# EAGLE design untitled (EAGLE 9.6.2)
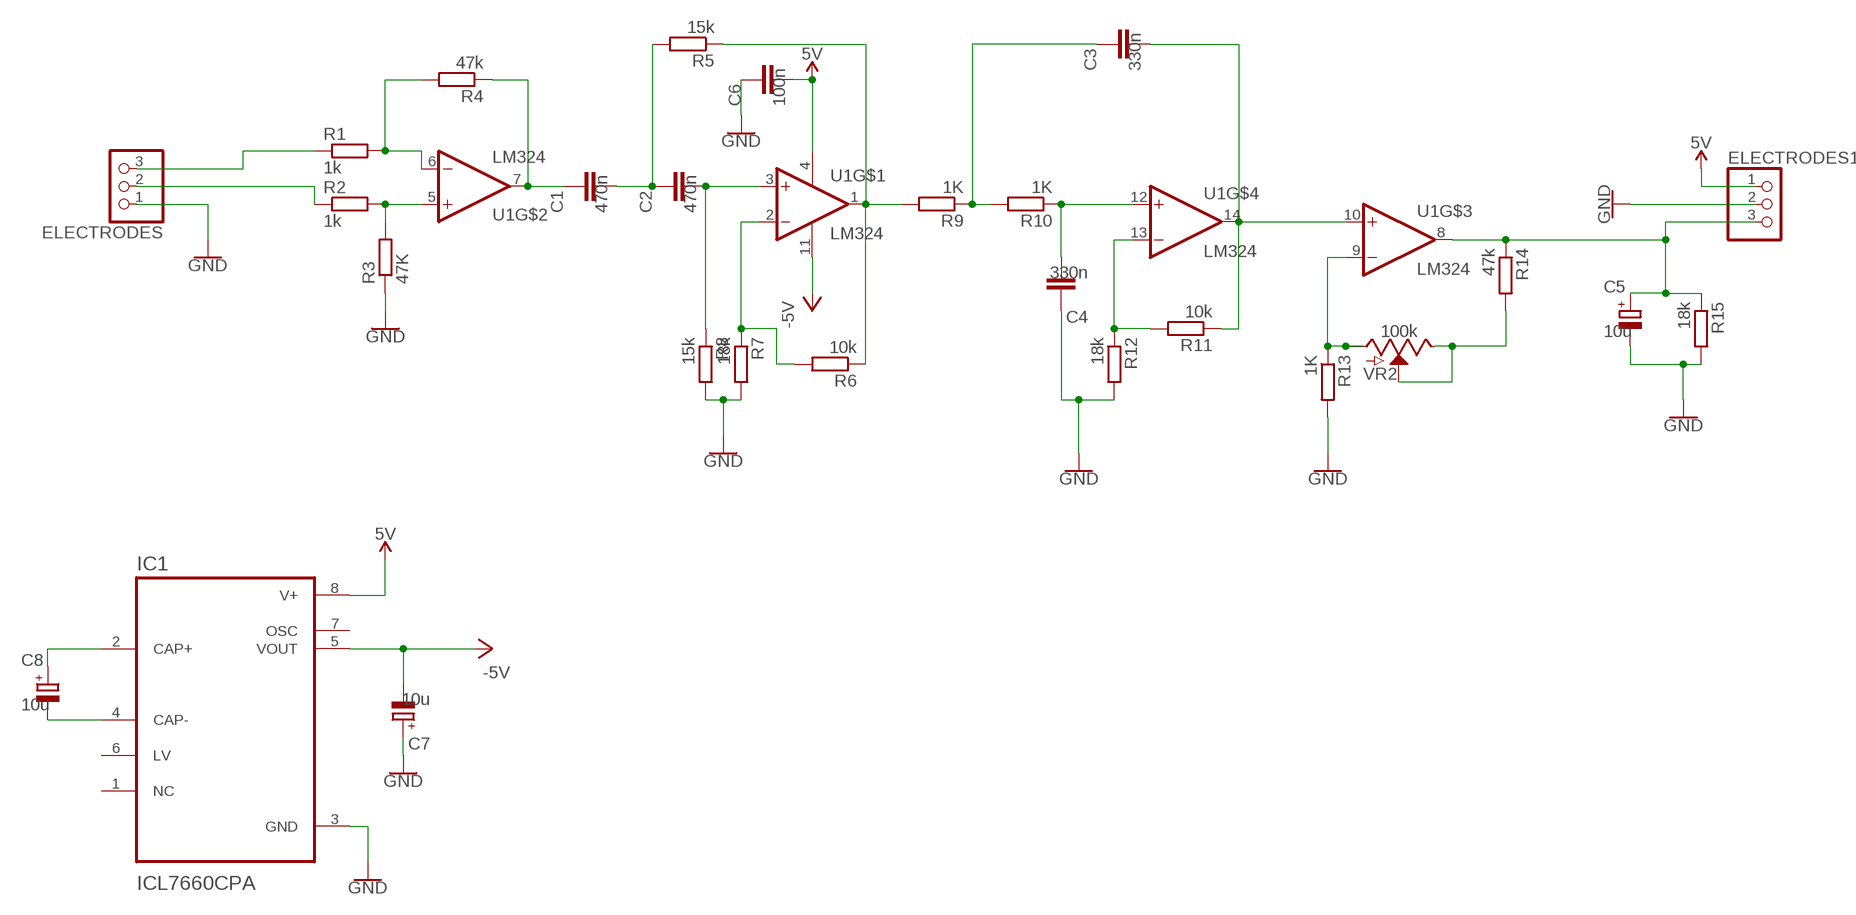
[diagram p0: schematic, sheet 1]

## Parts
C1  470n  C-EU025-024X044  [C025-024X044]
C2  470n  C-EU025-024X044  [C025-024X044]
C3  330n  C-EU025-024X044  [C025-024X044]
C4  330n  C-EU025-024X044  [C025-024X044]
C5  10u  CPOL-EUE2,5-6E  [E2,5-6E]
C6  100n  C-EU025-024X044  [C025-024X044]
C7  10u  CPOL-EUE2,5-6E  [E2,5-6E]
C8  10u  CPOL-EUE2,5-6E  [E2,5-6E]
ELECTRODES  PINHD-1X3  [1X03]
ELECTRODES1  PINHD-1X3  [1X03]
IC1  ICL7660CPA  [DIP794W47P254L991H457Q8]
R1  1k  R-EU_0204/7  [0204/7]
R2  1k  R-EU_0204/7  [0204/7]
R3  47K  R-EU_0204/7  [0204/7]
R4  47k  R-EU_0204/7  [0204/7]
R5  15k  R-EU_0204/7  [0204/7]
R6  10k  R-EU_0204/7  [0204/7]
R7  18k  R-EU_0204/7  [0204/7]
R8  15k  R-EU_0204/7  [0204/7]
R9  1K  R-EU_0204/7  [0204/7]
R10  1K  R-EU_0204/7  [0204/7]
R11  10k  R-EU_0204/7  [0204/7]
R12  18k  R-EU_0204/7  [0204/7]
R13  1K  R-EU_0204/7  [0204/7]
R14  47k  R-EU_0204/7  [0204/7]
R15  18k  R-EU_0204/7  [0204/7]
U1  LM324  [SOIC127P600X175-14N]
VR2  100k  POTENTIOMETER-PTH-9MM-1/20W-20%  [POT-PTH-ALPS]

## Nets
5V: C6.2 ELECTRODES1.1 IC1.8(V+) U1.4(VCC+)
-5V: C7.- IC1.5(VOUT) U1.11(VCC-)
GND: C4.1 C5.- C6.1 C7.+ ELECTRODES1.2 ELECTRODES.1 IC1.3(GND) R3.1 R7.2 R8.2 R12.2 R13.2 R15.2
N$1: ELECTRODES.3 R1.1
N$2: ELECTRODES.2 R2.1
N$3: R2.2 R3.2 U1.5(NON-INVERTING_INPUT2)
N$4: R1.2 R4.2 U1.6(INVERTING_INPUT2)
N$5: C1.1 R4.1 U1.7(OUTPUT2)
N$6: C1.2 C2.1 R5.2
N$7: C2.2 R8.1 U1.3(NON-INVERTING_INPUT1)
N$8: C3.1 R9.1 R10.2
N$9: R5.1 R6.1 R9.2 U1.1(OUTPUT1)
N$10: R6.2 R7.1 U1.2(INVERTING_INPUT1)
N$11: C4.2 R10.1 U1.12(NON-INVERTING_INPUT4)
N$12: R13.1 U1.9(INVERTING_INPUT3) VR2.P$3(A)
N$13: C3.2 R11.1 U1.10(NON-INVERTING_INPUT3) U1.14(OUTPUT4)
N$14: R14.2 VR2.P$1(E) VR2.P$2(S)
N$15: R11.2 R12.1 U1.13(INVERTING_INPUT4)
N$17: C5.+ ELECTRODES1.3 R14.1 R15.1 U1.8(OUTPUT3)
N$18: C8.- IC1.4(CAP-)
N$19: C8.+ IC1.2(CAP+)
Unconnected: IC1.1(NC) IC1.6(LV) IC1.7(OSC)

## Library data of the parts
C1-C4 C6 = rcl:C-EU: CAPACITOR, European symbol; SPICEPREFIX: C
C5 C7 C8 = rcl:CPOL-EU: POLARIZED CAPACITOR, European symbol; SPICEPREFIX: C
ELECTRODES ELECTRODES1 = adafruit:PINHD-1X3: PIN HEADER
IC1 = ICL7660CPA:ICL7660CPA; AVAILABILITY: Unavailable; DESCRIPTION: Charge Pump Switching Regulator IC Positive or Negative Fixed -Vin, 2Vin 1 Output 45mA 8-DIP (0.300, 7.62mm); DIGIKEY-PURCHASE-URL: https://snapeda.com/shop?store=DigiKey&id=184409; MF: Renesas Electronics; MP: ICL7660CPA; PACKAGE: DIP-8 Intel; PRICE: None
R1-R15 = rcl:R-EU_: RESISTOR, European symbol; SPICEPREFIX: R
U1 = LM324:LM324: these devices consist of four independent high-gain frequency-compensated operational amplifiers that are designed sp...; DESCRIPTION: General Purpose Amplifier 4 Circuit 14-SOIC; MF: Texas Instruments; MP: LM324; PACKAGE: SOIC-14 Texas Instruments
VR2 = SparkFun-Resistors:POTENTIOMETER: Potentiometer (Pot) Three-terminal potentiometers, with an adjustable wiper and two adjustable resistors. A pot can be used to create a configurable voltage divider, or as a variable resistor. Variants ALPS_POT and ALPS_POT_KIT - PTH, breadboard compatible, 9mm square pots Rotary Potentiometer -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; PROD_ID: RES-09177; SF_SKU: COM-09288; VALUE: 10k

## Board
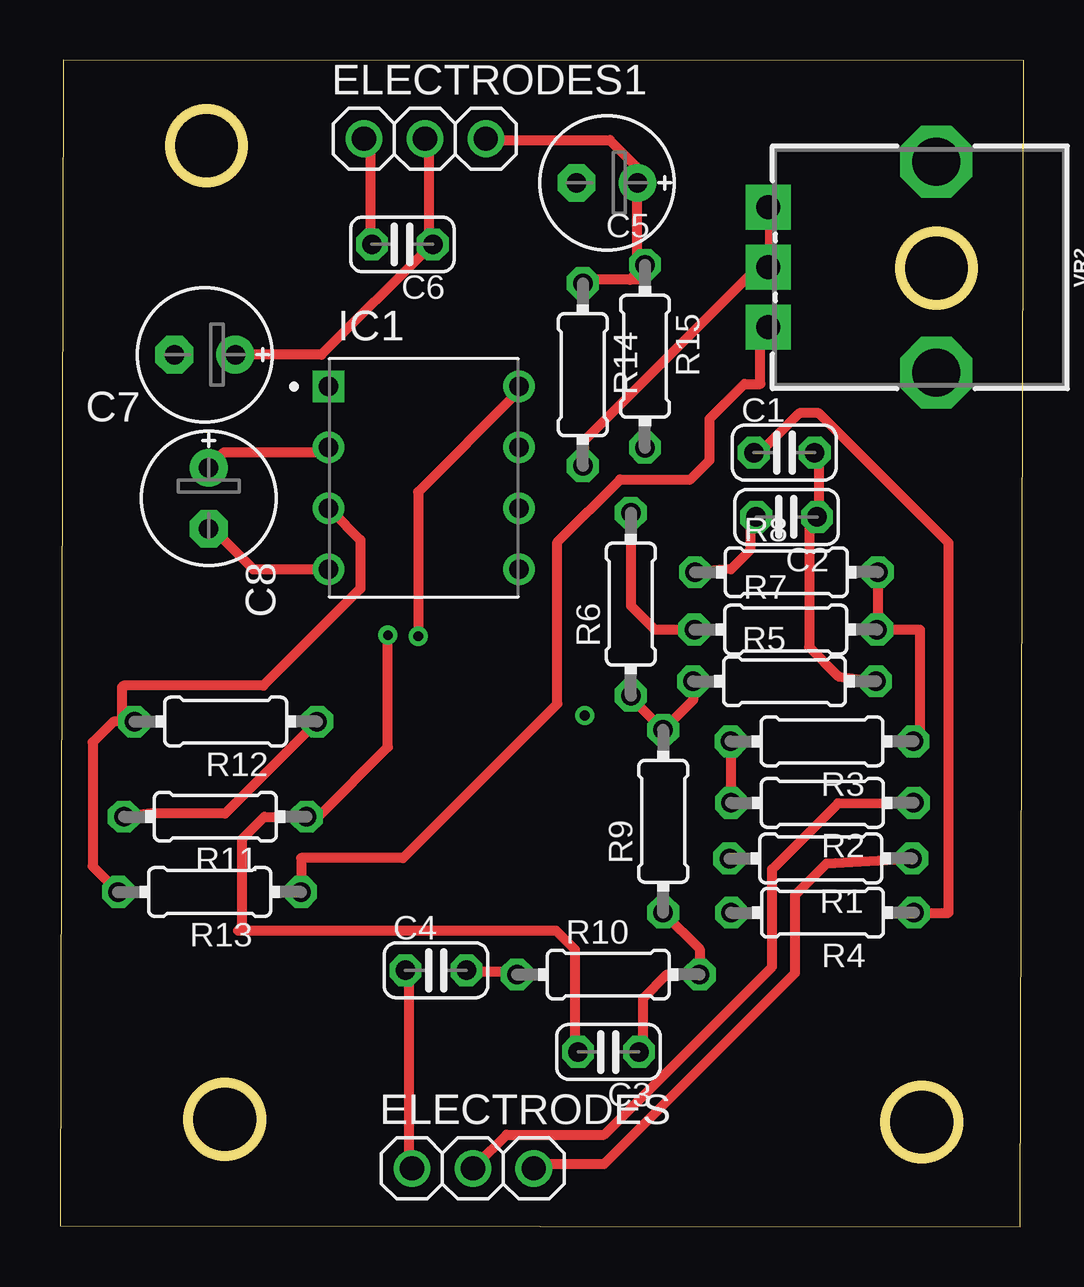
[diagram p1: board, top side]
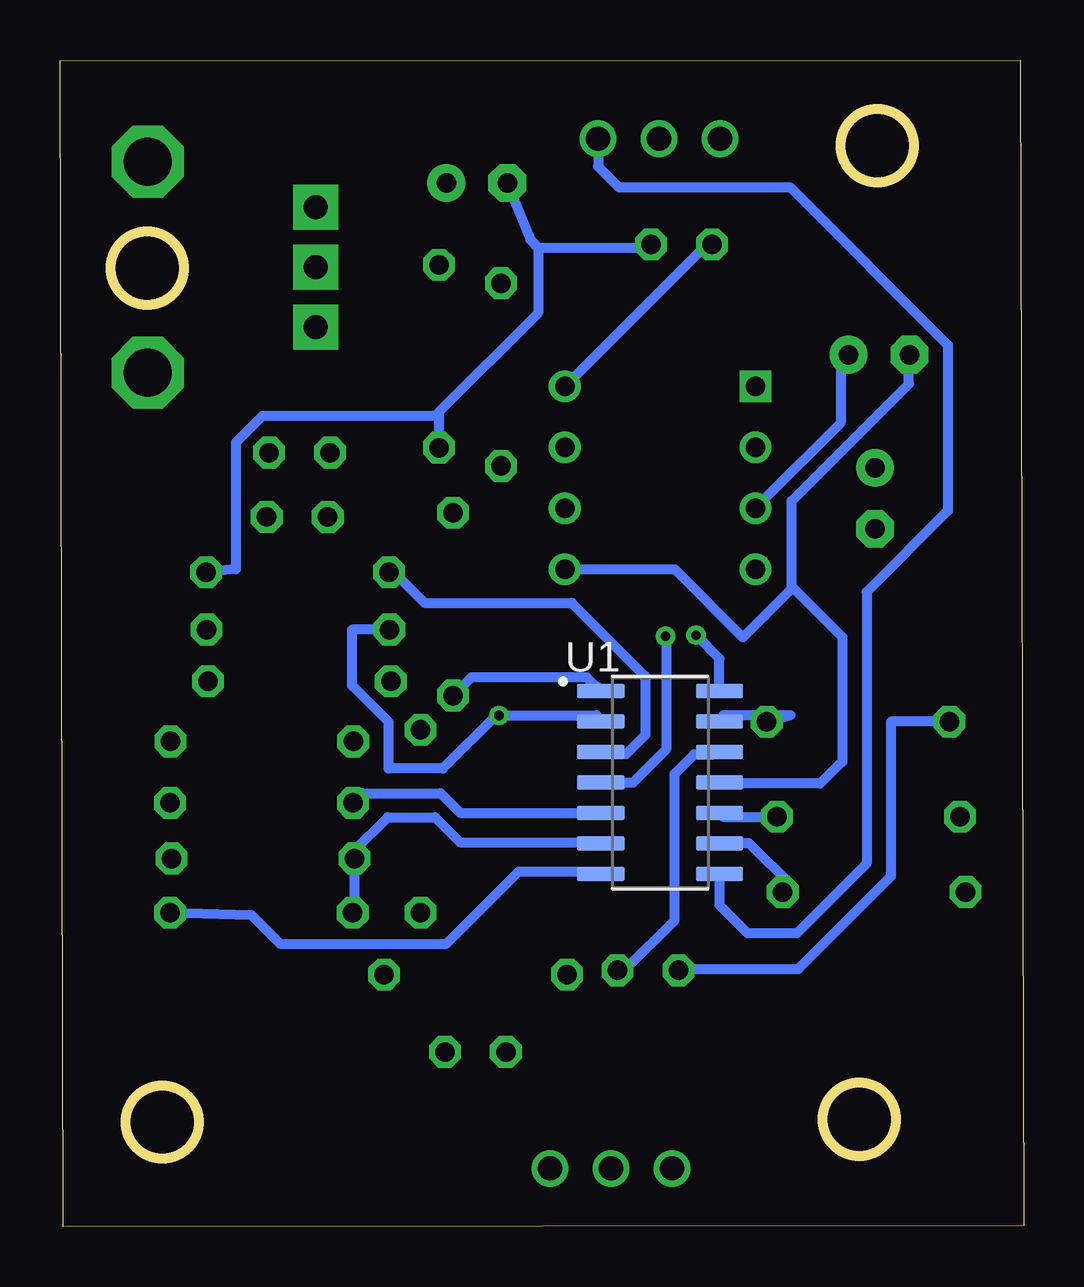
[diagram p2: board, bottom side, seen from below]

Size 40.16 x 48.63 mm. Coordinates in mm from the lower left corner, seen from the top.
Outline: 0,0.03 40.01,0 40.16,48.59 0.14,48.63 0,0.03
Outline: circle at 6.86,4.48 radius 1.52
Outline: circle at 35.91,4.36 radius 1.52
Outline: circle at 6.1,45.06 radius 1.52
Outline: circle at 36.52,39.95 radius 1.52
Copper layers (1*16): Top 0.035mm / dielectric 1.5mm / Bottom 0.035mm
Design rules "default *": minimum track width 16mil, minimum drill 0.4mm, track to track 16mil, track to pad 16mil, pad to pad 16mil, via to via 16mil, smd to smd 16mil, copper to edge 40mil, drill to drill 6mil, minimum pad ring 10mil, minimum via ring 8mil, stop-mask expansion 4mil, vias tented up to drill 0mil, thermal gap 10mil

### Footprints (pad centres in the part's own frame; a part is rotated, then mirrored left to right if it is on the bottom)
C025-024X044 = drill 0.813 octagon: 1 -1.27,0; 2 1.27,0
E2,5-6E = drill 0.813 pad 1.575: + -1.27,0 | drill 0.813 pad 1.575 octagon: - 1.27,0
1X03 = drill 1.016: 1 -2.54,0; 2 0,0; 3 2.54,0
DIP794W47P254L991H457Q8 = drill 0.81 pad 1.22 square: 1 -3.97,3.81 | drill 0.81 pad 1.22: 2 -3.97,1.27; 3 -3.97,-1.27; 4 -3.97,-3.81; 5 3.97,-3.81; 6 3.97,-1.27; 7 3.97,1.27; 8 3.97,3.81
0204/7 = drill 0.813 octagon: 1 -3.81,0; 2 3.81,0
SOIC127P600X175-14N = smd 1.97 x 0.6: 1 -2.475,3.81; 2 -2.475,2.54; 3 -2.475,1.27; 4 -2.475,0; 5 -2.475,-1.27; 6 -2.475,-2.54; 7 -2.475,-3.81; 8 2.475,-3.81; 9 2.475,-2.54; 10 2.475,-1.27; 11 2.475,0; 12 2.475,1.27; 13 2.475,2.54; 14 2.475,3.81
POT-PTH-ALPS = drill 1 pad 1.88 square: P$1 7,-2.5; P$2 7,0; P$3 7,2.5 | drill 2 octagon: P$4 0,-4.4; P$5 0,4.4

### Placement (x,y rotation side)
C1  30.18,32.26 0 top
C2  30.28,29.58 180 top
C3  22.85,7.28 180 top
C4  15.66,10.68 0 top
C5  22.79,43.51 180 top
C6  14.27,40.94 180 top
C7  6.03,36.34 180 top
C8  6.2,30.36 270 top
ELECTRODES  17.2,2.43 0 top
ELECTRODES1  15.2,45.35 0 top
IC1  15.16,31.21 0 top
R1  31.7,15.35 180 top
R2  31.76,17.66 180 top
R3  31.75,20.23 180 top
R4  31.77,13.08 180 top
R5  30.19,22.73 0 top
R6  23.78,25.95 90 top
R7  30.24,24.89 0 top
R8  30.26,27.28 0 top
R9  25.13,16.9 90 top
R10  22.84,10.51 0 top
R11  6.47,17.09 180 top
R12  6.9,21.05 180 top
R13  6.24,13.95 180 top
R14  21.78,35.51 270 top
R15  24.37,36.28 270 top
U1  15.16,18.51 0 bottom
VR2  36.51,39.99 180 top

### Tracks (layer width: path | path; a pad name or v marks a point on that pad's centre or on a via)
5V  (via drill 0.4)
  Top 0.406: C6.2 12.92,41.22 12.92,45.29 ELECTRODES1.1 | v14.93,24.6 v14.92,24.61 14.92,30.62 19.02,34.72 IC1.8
  Bottom 0.406: v14.93,24.6 14.93,24.45 14.9,24.42 14.9,19.89 16.28,18.51 U1.4 | C6.2 13.33,40.81 19.02,35.13 IC1.8
-5V
  Bottom 0.406: IC1.5 14.55,27.4 11.7,24.56 10.81,25.45 | U1.11 12.51,18.46 8.49,18.46 7.56,19.39 7.56,24.57 9.63,26.64 10.81,25.45 | 10.81,25.45 9.67,26.59 9.67,30.25 4.79,35.13 4.79,35.94 C7.-
GND
  Top 0.406: C4.1 14.55,10.33 14.55,2.61 ELECTRODES.1 | R8.2 34.07,24.91 R7.2 35.83,24.89 35.83,20.51 35.4,20.09 35.42,20.09 R3.1 | ELECTRODES1.2 15.36,45.29 15.36,41.22 C6.1 15.36,40.81 10.89,36.34 7.64,36.34 C7.+ | 2.94,21.05 R12.2 2.58,21.05 | IC1.3 11.3,29.84 12.51,28.62 12.51,26.59 8.48,22.55 2.65,22.55 2.58,22.48 2.58,21.05 | R13.2 1.36,15.02 1.36,20.18 2.23,21.05 2.58,21.05
  Bottom 0.406: R12.2 5.52,21.05 5.52,14.62 9.4,10.74 14.14,10.74 C4.1 | IC1.3 10.89,30.25 7.64,33.5 7.64,35.94 C7.+ | 20.24,40.81 20.24,38.08 24.37,33.95 R15.2 24.37,33.79 31.73,33.79 32.83,32.69 32.83,27.4 R8.2 | 20.24,40.81 20.55,41.13 C5.- | 20.24,40.81 15.77,40.81 C6.1
N$1
  Top 0.406: R1.1 31.95,15.14 30.63,13.82 30.63,10.57 22.67,2.61 19.83,2.61 ELECTRODES.3
N$2
  Top 0.406: R2.1 32.43,17.65 29.67,14.89 29.67,10.83 22.67,3.83 18.61,3.83 17.39,2.61 ELECTRODES.2
N$3
  Top 0.406: R3.2 27.95,20.21 R2.2
  Bottom 0.406: U1.5 23.49,17.24 24.3,18.06 27.56,18.06 R2.2
N$4
  Bottom 0.406: R4.2 27.89,13.16 R1.2 27.89,15.62 27.94,15.64 26.51,17.06 24.53,17.06 23.49,16.02 17.8,16.02 U1.6
N$5
  Top 0.406: R4.1 37.03,13.08 37.03,28.5 31.62,33.91 30.8,33.91 29.18,32.28 C1.1
  Bottom 0.406: U1.7 17.8,14.81 21.05,14.81 24.07,11.79 30.98,11.79 32.17,12.98 R4.1
N$6
  Top 0.406: C1.2 31.62,31.87 31.62,29.84 C2.1 31.21,29.44 31.21,24.15 32.43,22.93 R5.2
N$7
  Top 0.406: C2.2 28.77,29.44 28.77,28.22 27.96,27.4 R8.1
  Bottom 0.406: R8.1 26.25,27.28 24.97,26 18.83,26 15.77,22.93 15.77,20.49 16.58,19.68 17.39,19.68 U1.3
N$8
  Top 0.406: C3.1 24.3,7.49 24.3,9.52 25.29,10.51 R10.2 26.65,11.57 R9.1
N$9
  Top 0.406: 26.81,22.8 R5.1 26.38,21.95 R9.2 23.78,22.06 R6.1
  Bottom 0.406: 17.8,22.53 U1.1 18.21,22.9 23.02,22.9 R6.1
N$10  (via drill 0.4)
  Top 0.406: 26.37,24.92 26.4,24.92 R7.1 24.78,24.89 23.78,25.88 R6.2
  Bottom 0.406: U1.2 17.8,21.31 v21.86,21.31 21.99,21.31 24.2,19.09 26.47,19.09 26.47,21.03 27.99,22.55 27.99,24.89 R7.1
N$11
  Top 0.406: C4.2 17,10.61 19.08,10.61 19.03,10.57 R10.1
  Bottom 0.406: U1.12 12.92,19.68 13.73,19.68 14.55,18.87 14.55,12.77 16.58,10.74 C4.2
N$12
  Top 0.406: R13.1 10.05,15.37 14.29,15.37 20.72,21.79 20.72,28.53 23.34,31.15 26.27,31.15 27.06,31.94 27.06,33.68 28.51,35.13 29.18,35.13 29.18,37.16 VR2.P$3
  Bottom 0.406: U1.9 12.66,15.98 11.45,15.98 9.57,14.11 R13.1
N$13  (via drill 0.4)
  Top 0.406: R11.1 10.76,17.09 13.66,19.99 v13.66,24.66 | 7.42,12.35 7.58,12.35 | 7.58,12.35 20.66,12.35 21.46,11.55 21.46,7.49 C3.2 | 10.63,17.1 10.61,17.09 R11.1 | 7.58,12.35 7.58,16.16 8.51,17.09 R11.1
  Bottom 0.406: v13.66,24.66 12.68,23.68 U1.14 | U1.10 12.52,17.09 R11.1
N$14
  Top 0.406: R14.2 21.82,31.74 21.82,32.74 29.09,40.01 VR2.P$2 29.58,40 29.58,42.44 VR2.P$1
N$15
  Top 0.406: R11.2 3.8,17.22 6.88,17.22 R12.1
  Bottom 0.406: U1.13 12.51,21.31 9.71,21.31 R12.1
N$17
  Top 0.406: 24.34,39.47 23.75,39.47 | 23.75,39.47 21.93,39.47 R14.1 | 24.34,43.4 C5.+ | C5.+ 24.06,44.14 22.91,45.29 17.8,45.29 ELECTRODES1.3 | 23.75,39.47 R15.1 24.06,40.4 C5.+
  Bottom 0.406: U1.8 12.68,13.4 11.51,12.23 9.46,12.23 6.55,15.14 6.55,26.46 3.17,29.84 3.17,36.75 9.74,43.32 16.88,43.32 17.74,44.18 ELECTRODES1.3
N$18
  Top 0.406: IC1.4 8.04,27.4 6.42,29.03 C8.-
N$19
  Top 0.406: IC1.2 10.89,32.28 6.83,32.28 6.42,31.87 C8.+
